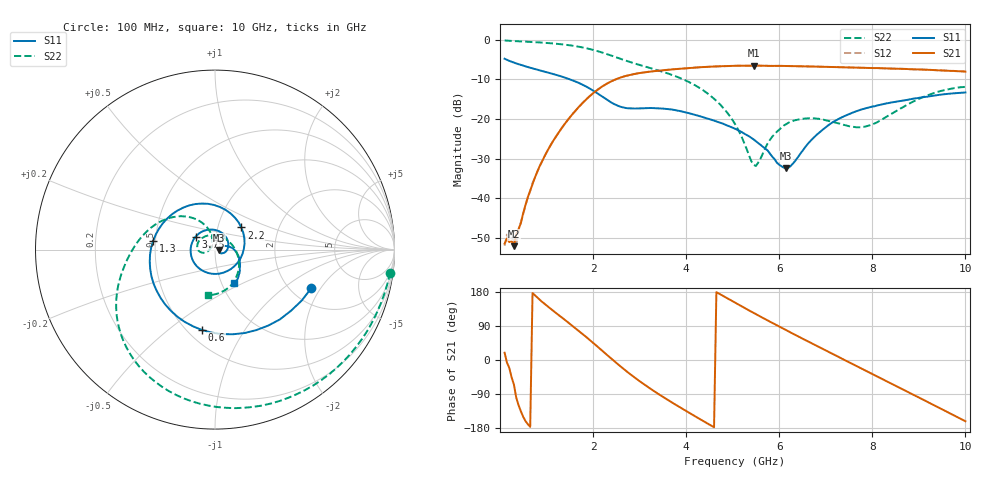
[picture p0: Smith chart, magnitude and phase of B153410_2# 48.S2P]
!  2-Port S-parameters saved by WinCal
! VAR MeasName=S-Parameters (CALIBRATED_DATA) read from VNA (N5245A)
! VAR MeasDate=2016-12-23 10:01:50
! VAR NAME=B153410_2# 48
! VAR FILENAME=B153410_2# 48.S2P
! VAR DATE=2016-12-23 10:01:50
! VAR PHYS_PORTS=1,2
# Hz S DB R 50
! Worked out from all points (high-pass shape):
!   199 points, 100 MHz to 10 GHz, reference 50 ohm
!   highest |S21| = -6.50 dB at 5.45 GHz (marker M1); lowest = -52.2 dB at 300 MHz (marker M2)
!   |S21| within 3 dB of the highest: 2.593 GHz to end of sweep
!   lowest |S11| = -32.4 dB at 6.15 GHz (marker M3), VSWR 1.05, Z = 52.4 - j0.216 ohm
!   |S11| at or under -10 dB: 1.509 GHz to end of sweep
!   |S22| runs from -31.9 to -0.1 dB; largest |S21 - S12| = 0.0034
!   S11 on the Smith chart (normalised r, x): 100 MHz: 2.56, -1.65; 600 MHz: 0.59, -0.66; 1.3 GHz: 0.49, +0.05; 2.2 GHz: 1.30, +0.33; 3.75 GHz: 0.80, +0.12; 10 GHz: 1.14, -0.45
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1e8  -4.76 -21.7  -51.51 19.3  -52.07 27.4  -0.13 -7.5
1.5e8  -5.03 -30.5  -50.22 -6.7  -49.25 -0.2  -0.18 -11.0
3e8  -5.73 -55.0  -52.17 -64.9  -50.79 -74.2  -0.28 -21.0
3.5e8  -5.95 -62.8  -49.13 -99.2  -51.90 -89.4  -0.31 -24.3
4e8  -6.14 -70.4  -47.83 -119.4  -48.09 -115.9  -0.33 -27.6
6e8  -6.86 -99.0  -39.73 -169.6  -39.87 -169.4  -0.45 -40.8
9.5e8  -8.01 -144.8  -29.63 149.2  -29.63 149.0  -0.71 -63.5
1.3e9  -9.16 172.0  -22.76 115.0  -22.75 115.0  -1.07 -85.9
1.75e9  -11.18 113.1  -16.25 71.1  -16.27 71.1  -1.84 -114.2
2.2e9  -14.35 40.0  -11.75 24.1  -11.77 24.3  -3.20 -140.5
2.75e9  -17.29 -70.5  -8.98 -32.8  -8.97 -32.5  -5.41 -165.9
3.4e9  -17.30 -172.1  -7.80 -89.3  -7.76 -89.3  -7.71 169.4
3.75e9  -17.72 146.6  -7.41 -116.2  -7.40 -116.2  -9.08 155.1
4.45e9  -19.84 70.8  -6.80 -166.9  -6.81 -166.9  -13.44 124.6
5.05e9  -22.46 12.0  -6.54 151.3  -6.56 151.4  -21.26 104.3
5.45e9  -25.17 -18.1  -6.50 124.3  -6.52 124.4  -31.59 141.4
6.15e9  -32.41 -4.9  -6.59 78.7  -6.60 78.7  -21.28 -172.7
6.7e9  -25.19 20.4  -6.71 43.8  -6.72 43.9  -19.80 157.8
7.5e9  -18.78 -4.6  -6.94 -5.9  -6.96 -5.9  -21.83 95.2
8.35e9  -15.97 -29.2  -7.24 -58.7  -7.21 -58.4  -19.12 2.7
9.15e9  -14.41 -44.8  -7.52 -108.4  -7.53 -108.3  -14.19 -53.5
1e10  -13.29 -60.4  -8.00 -161.5  -8.00 -161.2  -11.86 -98.5
